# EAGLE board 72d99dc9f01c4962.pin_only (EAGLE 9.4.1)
REV: A

Size 35.56 x 33.02 mm. Coordinates in mm from the lower left corner, seen from the top.
Outline: 0,30.48 0,2.54 arc90 2.54,0 arc90 5.08,2.54 5.08,5.08 30.48,5.08 30.48,2.54 arc90 33.02,0 arc90 35.56,2.54 35.56,30.48 arc90 33.02,33.02 2.54,33.02 arc90 0,30.48
Copper layers (1*16): Top 0.035mm / dielectric 1.5mm / Bottom 0.035mm
Design rules "adafruit *": minimum track width 8mil, minimum drill 15.5mil, track to track 8mil, track to pad 8mil, pad to pad 8mil, via to via 8mil, smd to smd 8mil, copper to edge 10mil, drill to drill 8mil, minimum pad ring 10mil, minimum via ring 8mil, stop-mask expansion 2mil, vias tented up to drill 20mil, thermal gap 10mil

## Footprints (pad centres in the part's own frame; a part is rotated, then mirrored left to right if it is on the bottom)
0603-NO = smd 1.075 x 1: 1 -0.85,0; 2 0.85,0
0805-NO = smd 1.24 x 1.5: 1 -0.95,0; 2 0.95,0
JST_SH4 = smd 0.6 x 1.55: 1 -1.5,2.514; 2 -0.5,2.514; 3 0.5,2.514; 4 1.5,2.514 | smd 1.2 x 1.8: MT1 -2.8,-1.386; MT2 2.8,-1.386
CHIPLED_0603_NOOUTLINE = smd 0.8 x 0.8: A 0,-0.75; C 0,0.75
SOD-323 = smd 1.35 x 0.8: A 1.27,0; C -1.27,0
FIDUCIAL_1MM = smd 1 x 1: 1 0,0
SOT23 = smd 1 x 1.4: 1 -0.95,-1.1; 2 0.95,-1.1; 3 0,1.1
1X08_ROUND_70 = drill 1 pad 1.778: 1 -8.89,0; 2 -6.35,0; 3 -3.81,0; 4 -1.27,0; 5 1.27,0; 6 3.81,0; 7 6.35,0; 8 8.89,0
SOT363 = smd 0.5 x 0.5: 1 -0.75,-0.9; 3 0.75,-0.9; 4 0.75,0.9; 6 -0.75,0.9 | smd 0.4 x 0.5: 2 0,-0.9; 5 0,0.9
RESPACK_4X0603 = smd 0.45 x 0.9: 1 -1.3,-0.85; 2 -0.4,-0.85; 3 0.4,-0.85; 4 1.3,-0.85; 5 1.3,0.85; 6 0.4,0.85; 7 -0.4,0.85; 8 -1.3,0.85
SOLDERJUMPER_CLOSEDWIRE = smd 1.168 x 1.6: 1 -0.762,0; 2 0.762,0 | smd 0.635 x 0.203: WIRE 0,0
SOLDERJUMPER_ARROW_NOPASTE = smd 0.762 x 1.524: 1 -1.016,0; 2 1.016,0
UG-2864HSWEG01_1.3_WRAPAROUND = smd 0.35 x 2.2 bottom: 1 -10.15,-0.2; 2 -9.45,-0.2; 3 -8.75,-0.2; 4 -8.05,-0.2; 5 -7.35,-0.2; 6 -6.65,-0.2; 7 -5.95,-0.2; 8 -5.25,-0.2; 9 -4.55,-0.2; 10 -3.85,-0.2; 11 -3.15,-0.2; 12 -2.45,-0.2; 13 -1.75,-0.2; 14 -1.05,-0.2; 15 -0.35,-0.2; 16 0.35,-0.2; 17 1.05,-0.2; 18 1.75,-0.2; 19 2.45,-0.2; 20 3.15,-0.2; 21 3.85,-0.2; 22 4.55,-0.2; 23 5.25,-0.2; 24 5.95,-0.2; 25 6.65,-0.2; 26 7.35,-0.2; 27 8.05,-0.2; 28 8.75,-0.2; 29 9.45,-0.2; 30 10.15,-0.2 | hole 0.4: -8,-4.45; 8,-4.45
SOT23-5 = smd 0.55 x 1.2: 1 -0.95,-1.3; 2 0,-1.3; 3 0.95,-1.3; 4 0.95,1.3; 5 -0.95,1.3
MOUNTINGHOLE_2.5_PLATED = drill 2.5 pad 3.2: P$1 0,0

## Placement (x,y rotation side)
C1  0.1uF  [0603-NO]  10.41,24.89 90 top
C2  10uF  [0805-NO]  2.54,24.77 270 top
C3  10uF  [0805-NO]  8.38,24.64 90 top
C12  2.2uF  [0805-NO]  27.36,18.1 90 top
C13  2.2uF  [0805-NO]  24.95,18.1 90 top
C14  10uF  [0805-NO]  7.75,16.03 270 top
C15  10uF  [0805-NO]  23.04,18.1 270 top
C16  10uF  [0805-NO]  9.65,16.03 270 top
C17  1uF  [0603-NO]  21.38,18.1 270 top
CONN1  STEMMA_I2C_QT  [JST_SH4]  33.02,16.51 90 top
CONN4  STEMMA_I2C_QT  [JST_SH4]  2.54,16.51 270 top
D1  GREEN  [CHIPLED_0603_NOOUTLINE]  2.03,11.68 90 top
D3  1N4148  [SOD-323]  14.99,24.79 270 top
D4  1N4148  [SOD-323]  18.57,25.53 180 top
D5  1N4148  [SOD-323]  22.35,24.41 270 top
FID3  FIDUCIAL_1MM  [FIDUCIAL_1MM]  2.29,7.94 0 top
FID4  FIDUCIAL_1MM  [FIDUCIAL_1MM]  33.78,25.82 0 top
IC5  APX803  [SOT23]  16,19.94 0 top
JP2  [1X08_ROUND_70]  17.78,30.48 180 top
Q2  BSS138  [SOT363]  25.65,23.88 90 top
R1  10K  [0603-NO]  2.29,10.16 0 top
R2  10K  [RESPACK_4X0603]  18.8,21.84 180 top
R3  10K  [RESPACK_4X0603]  29.84,24.26 90 top
R9  390K  [0603-NO]  11.3,16.03 270 top
SJ1  [SOLDERJUMPER_CLOSEDWIRE]  13.09,20.7 270 top
SJ2  [SOLDERJUMPER_CLOSEDWIRE]  10.77,20.7 270 top
SJ3  [SOLDERJUMPER_ARROW_NOPASTE]  23.5,21.21 180 top
U1  UG-2864HSWEG01  [UG-2864HSWEG01_1.3_WRAPAROUND]  17.78,12.57 0 bottom
U2  AP2112K-3.3  [SOT23-5]  5.33,24.51 180 top
U$1  MOUNTINGHOLE2.5  [MOUNTINGHOLE_2.5_PLATED]  2.54,30.48 0 top
U$8  [ADAFRUIT_5MM]  30.23,7.87 0 top
U$17  MOUNTINGHOLE2.5  [MOUNTINGHOLE_2.5_PLATED]  33.02,30.48 0 top
U$19  MOUNTINGHOLE2.5  [MOUNTINGHOLE_2.5_PLATED]  2.54,2.54 0 top
U$21  MOUNTINGHOLE2.5  [MOUNTINGHOLE_2.5_PLATED]  33.02,2.54 0 top
U$25  [PCBFEAT-REV-040]  32.64,6.86 0 top
U$31  [STEMMAQT]  0.25,19.81 0 top

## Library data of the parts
C1-C3 C12-C17 CONN1 CONN4 D1 D3-D5 JP2 Q2 R1-R3 R9 SJ1 SJ2 U2 U$8 U$25 = microbuilder
FID3 FID4 SJ3 U$1 U$17 U$19 U$21 = microbuilder; BOM: EXCLUDE
IC5 = adafruit
U1 = adafruit_display
U$31 = silks

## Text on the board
tPlace: GND | 3Vo | Rst | A0 | Clk | VIN | CS | DC | Data | 1.3" 128x64 OLED Display | A0 | I2C / Addr / 0x3D | J1 | J2 | Bus default is I2C / For SPI open J1/J2 | on
bPlace: GND | 3Vo | Rst | A0 | Clk | VIN | CS | DC | Data

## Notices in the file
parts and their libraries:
microbuilder: This work is placed in the public domain, and may be freely used for commercial and non-commercial work with the following conditions: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
